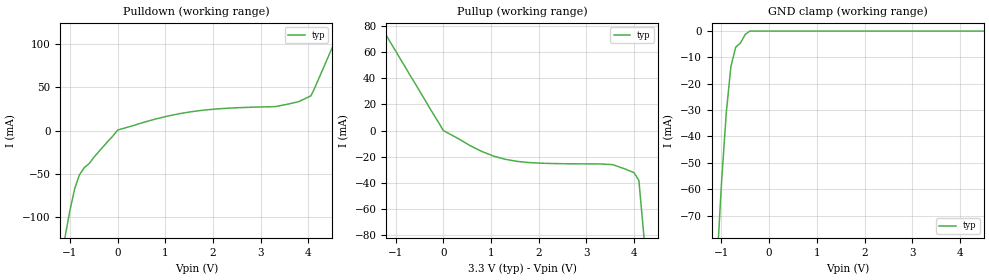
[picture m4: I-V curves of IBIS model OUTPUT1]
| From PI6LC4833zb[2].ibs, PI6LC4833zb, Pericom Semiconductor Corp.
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|   Model OUTPUT1 (CMOS)
[Model] OUTPUT1
Model_type Output
Vref =  0.000V
Vmeas = 1.650V
| variable   typ   min   max
C_comp   4.300pF  NA   NA
[Voltage Range]   3.300V   NA   NA
[GND Clamp Reference]   0.000V   NA   NA
[POWER Clamp Reference]   3.300V   NA   NA
[Pullup Reference]   3.300V   NA   NA
[Pulldown Reference]   0.000V   NA   NA
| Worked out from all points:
|   slope of the pulldown table from 0 to 0.495 V, typ, clamps not added: 61.6 ohm
|   slope of the pullup table from 0 to 0.495 V, typ, clamps not added: 49.1 ohm
|   GND clamp passes 1 mA (typ) near -0.48 V on its own axis
[GND Clamp]
| Voltage   I(typ)   I(min)   I(max)
-3.3V     -968.6mA   NA         NA
-1.101V   -91.06mA   NA         NA
-999.6mV  -58.06mA   NA         NA
-898.5mV  -31.14mA   NA         NA
-802.4mV  -13.62mA   NA         NA
-701.1mV  -6.13mA    NA         NA
-599.9mV  -4.51mA    NA         NA
-498.7mV  -1.21mA    NA         NA
-403mV    0A         NA         NA
6.602V    0A         NA         NA
[Pulldown]
| Voltage   I(typ)   I(min)   I(max)
-3.3V     -970.1mA   NA         NA
-1.101V   -122.5mA   NA         NA
-898.5mV  -66.74mA   NA         NA
-802.5mV  -51.44mA   NA         NA
0V        600uA      NA         NA
800mV     13.43mA    NA         NA
1.55V     21.86mA    NA         NA
3.3V      27.7mA     NA         NA
3.8V      33.56mA    NA         NA
4.05V     40.21mA    NA         NA
4.099V    45.33mA    NA         NA
6.602V    364.3mA    NA         NA
[Pullup]   |Note: Vtable = Vcc - Voutput
| Voltage   I(typ)   I(min) I(max)
-3.3V     222.2mA    NA         NA
-1.303V   79.54mA    NA         NA
0V        -60uA      NA         NA
550mV     -11.33mA   NA         NA
800mV     -15.9mA    NA         NA
1.05V     -19.47mA   NA         NA
1.55V     -23.57mA   NA         NA
2.05V     -24.93mA   NA         NA
3.55V     -26.05mA   NA         NA
3.998V    -32.17mA   NA         NA
4.099V    -38.16mA   NA         NA
6.603V    -1.056A    NA         NA
[POWER Clamp]   |Note: Vtable = Vcc - Voutput
| Voltage   I(typ)   I(min)  I(max)
-3.3V     0A         NA         NA
0V        0A         NA         NA
[Ramp]
| variable   typ   min   max
dV/dt_r   1V/500.00p   NA   NA
dV/dt_f   1V/520.00p   NA   NA
